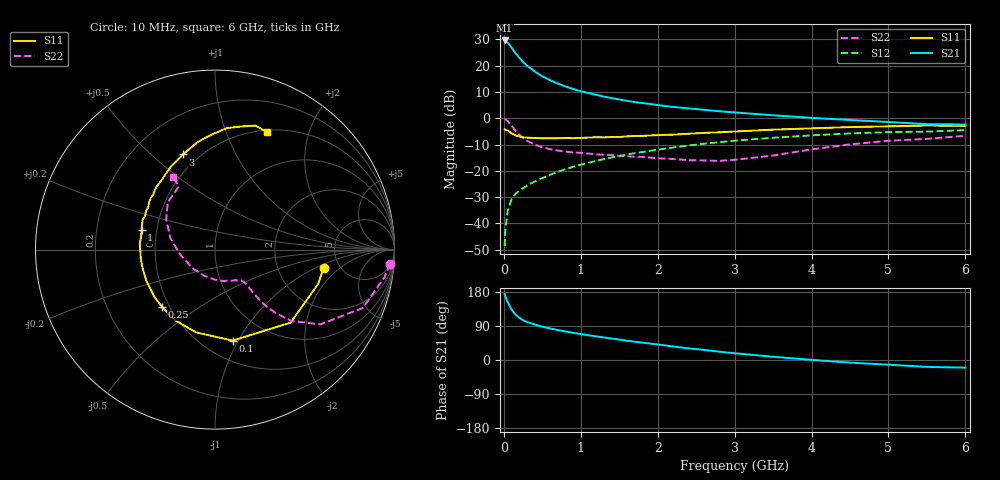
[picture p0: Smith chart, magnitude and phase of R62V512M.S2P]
! SIEMENS Small Signal Semiconductors
! BFR193
! Si NPN RF Bipolar Junction Transistor in SOT23
! VCE = 2.5 V  IC = 12 mA
! Common Emitter S-Parameters:  May  1996
# GHz  S  MA  R  50
!  f  S11  S21  S12  S22
! GHz  MAG  ANG  MAG  ANG  MAG  ANG  MAG  ANG
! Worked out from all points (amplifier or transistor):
!   36 points, 10 MHz to 6 GHz, reference 50 ohm
!   highest |S21| = 29.6 dB at 10 MHz (marker M1)
!   |S21| within 3 dB of that: start of sweep to 107.4 MHz
!   unconditionally stable (mu >= 1): 671.8 MHz to 1.886 GHz
!   at 250 MHz: K = 0.71, MSG = 24.0 dB, |S12| = -26.6 dB
!   at 1.4 GHz: K = 1.03, MAG = 10.2 dB, |S12| = -14.9 dB
!   at 6 GHz: K = 0.95, MSG = 1.1 dB, |S12| = -4.5 dB
!   S11 on the Smith chart (normalised r, x): 10 MHz: 3.76, -1.22; 100 MHz: 0.69, -0.95; 250 MHz: 0.46, -0.36; 1 GHz: 0.41, +0.11; 3 GHz: 0.41, +0.63; 6 GHz: 0.52, +1.40
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0.01  0.6139 -9.5  30.13 174.3  0.0037 85.5  0.9777 -4.6
0.02  0.6058 -18.4  29.74 168.4  0.0076 81.5  0.9572 -9.2
0.05  0.5855 -44.0  27.45 152.9  0.0173 72.8  0.8862 -21.5
0.1  0.5165 -79.0  22.1 133.3  0.0288 62.8  0.7196 -35.4
0.15  0.4732 -102.8  17.41 120.1  0.0365 57.4  0.5814 -43.1
0.2  0.4527 -119.6  14.18 111.6  0.0419 57.3  0.4879 -46.3
0.25  0.4346 -132.9  11.79 105.0  0.047 57.2  0.4197 -48.0
0.3  0.4283 -141.9  10.05 100.5  0.0523 58.7  0.3743 -48.5
0.4  0.4203 -155.6  7.755 93.8  0.0626 60.4  0.3165 -48.5
0.5  0.4167 -165.5  6.264 88.0  0.0728 62.0  0.2808 -48.2
0.6  0.4163 -173.0  5.299 83.3  0.0841 63.3  0.2584 -47.8
0.7  0.4167 -179.5  4.587 79.1  0.0954 64.1  0.2439 -48.2
0.8  0.4207 175.4  4.025 75.4  0.1072 64.2  0.2318 -49.1
1  0.4227 165.3  3.277 68.6  0.1306 64.0  0.2197 -51.1
1.1  0.4293 161.7  3.016 65.3  0.1427 63.8  0.2133 -53.4
1.6  0.4528 143.9  2.145 50.9  0.2038 60.1  0.1887 -66.1
2.2  0.4882 127.5  1.641 35.8  0.278 53.4  0.1681 -89.7
3  0.5596 108.7  1.291 17.8  0.3746 42.2  0.1623 -139.7
3.5  0.6074 99.1  1.139 8.5  0.4258 34.5  0.1953 -171.4
4.5  0.68 84.5  0.927 -6.9  0.5146 19.8  0.3189 148.6
5.5  0.7271 71.8  0.772 -18.2  0.5577 4.7  0.4054 119.9
6  0.7151 66.2  0.762 -20.2  0.5951 0.2  0.4639 120.0
